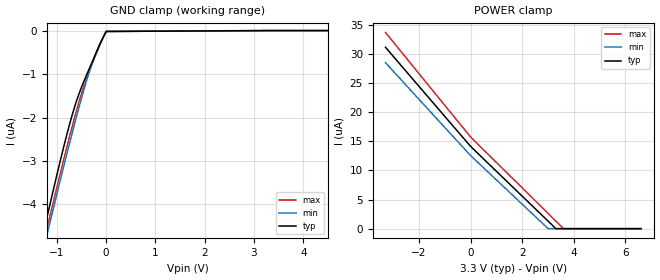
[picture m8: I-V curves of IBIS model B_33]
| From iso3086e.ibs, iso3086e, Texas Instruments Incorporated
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|   B_33 Model
[Model]   B_33
Model_type   Input
|Signals   B   negative pin
|Rref = 27   Note: 54 Ohm differential load;
Vinl   = 0.8
Vinh   = 2
| C_comp   obtained at 20MHz
|   typ   min   max
C_comp   5.326fF   5.258fF   5.400fF
[Voltage Range]   3.3   3   3.6
[Temperature Range]   40   125   -40
[Power Clamp Reference]   3.3   3   3.6
[GND Clamp Reference]   0   0   0
[GND Clamp]
|   Voltage   I(typ)   I(min)   I(max)
-3.3V     -15.09uA   -14.87uA   -15.56uA
-1.261V   -4.604uA   -4.989uA   -4.853uA
-1.201V   -4.31uA    -4.71uA    -4.568uA
-1.082V   -3.728uA   -4.155uA   -4.003uA
-864.6mV  -2.699uA   -3.152uA   -2.992uA
-735.9mV  -2.137uA   -2.573uA   -2.417uA
-627mV    -1.716uA   -2.096uA   -1.952uA
-458.7mV  -1.193uA   -1.396uA   -1.306uA
-285.4mV  -730.3nA   -768.8nA   -772.8nA
-117.2mV  -290.2nA   -282.6nA   -306.7nA
1.65mV    -20.02nA   -20.03nA   -19.91nA
6.6V      0A         0A         0A
[POWER Clamp]
|   Voltage   I(typ)   I(min)   I(max)
-3.3V     31.13uA    28.49uA    33.67uA
1.65mV    14.1uA     12.53uA    15.71uA
3.001V    1.289uA    0A         2.614uA
3.303V    0A         0A         1.296uA
3.6V      0A         0A         0A
6.6V      0A         0A         0A
